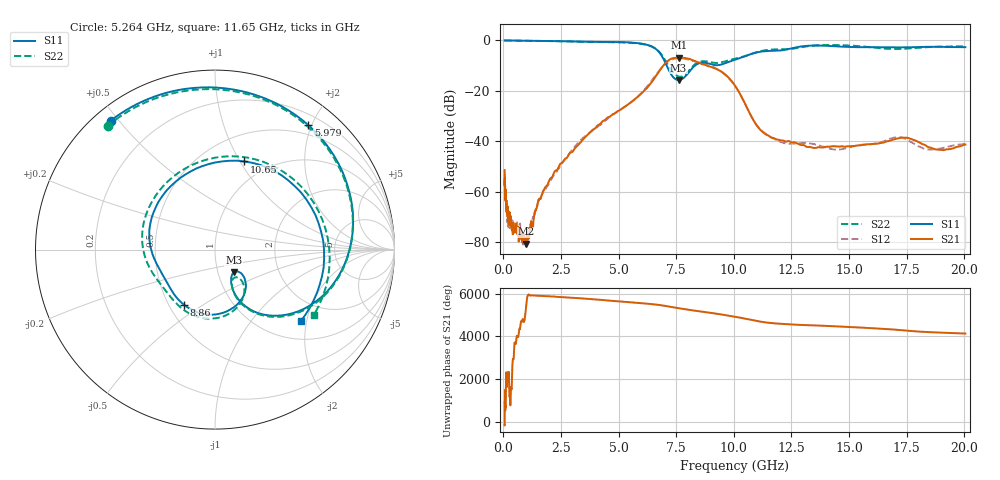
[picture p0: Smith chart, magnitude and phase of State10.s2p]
# Hz S DB R 50
!freq MagS11 AngS11 MagS21 AngS21 MagS12 AngS12 MagS22 AngS22
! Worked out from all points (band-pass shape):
!   1601 points, 50 MHz to 20.05 GHz, reference 50 ohm
!   highest |S21| = -6.83 dB at 7.627 GHz (marker M1); lowest = -80.7 dB at 979 MHz (marker M2)
!   |S21| within 3 dB of the highest: 6.951 GHz to 8.795 GHz (1.844 GHz wide, 23.4 % of centre)
!   lowest |S11| = -15.7 dB at 7.599 GHz (marker M3), VSWR 1.39, Z = 59.4 - j15.4 ohm
!   |S11| at or under -10 dB: 7.084 GHz to 8.309 GHz (1.225 GHz wide, 15.9 % of centre)
!   |S22| runs from -14.4 to 0.0 dB; largest |S21 - S12| = 0.025
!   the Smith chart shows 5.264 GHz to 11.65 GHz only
!   S11 on the Smith chart (normalised r, x): 5.264 GHz: 0.05, +0.48; 5.979 GHz: 0.35, +1.95; 8.86 GHz: 0.60, -0.42; 10.65 GHz: 0.78, +1.04; 11.65 GHz: 1.42, -1.84
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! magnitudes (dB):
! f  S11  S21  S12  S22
! 50 MHz  0.0  -51.5  -53.5  0.0
! 61.9 MHz  0.0  -55.4  -62.0  0.0
! 80.76 MHz  0.0  -60.7  -59.2  0.0
! 135.9 MHz  0.0  -67.6  -66.9  0.0
! 216.3 MHz  0.0  -70.5  -72.9  0.0
! 369.6 MHz  0.0  -74.2  -73.5  0.0
! 730.9 MHz  -0.1  -78.0  -74.1  -0.1
! 979 MHz  -0.1  -80.7  -81.6  -0.1
! 1.005 GHz  -0.1  -80.2  -81.6  -0.1
! 2.722 GHz  -0.3  -46.8  -46.6  -0.4
! 5.264 GHz  -0.7  -26.3  -26.3  -0.8
! 5.979 GHz  -1.2  -21.1  -21.0  -1.3
! 6.69 GHz  -4.0  -13.2  -12.8  -3.9
! 7.402 GHz  -14.9  -7.0  -7.3  -13.1
! 7.599 GHz  -15.7  -6.8  -7.1  -14.3
! 7.627 GHz  -15.7  -6.8  -7.1  -14.4
! 8.86 GHz  -9.1  -10.1  -9.8  -8.4
! 9.803 GHz  -8.4  -15.1  -15.3  -7.8
! 10.65 GHz  -5.7  -28.1  -28.1  -5.7
! 11.65 GHz  -4.1  -38.6  -38.6  -3.6
! 14.42 GHz  -2.3  -42.1  -43.3  -1.8
! 20.05 GHz  -2.7  -41.3  -41.0  -2.3
